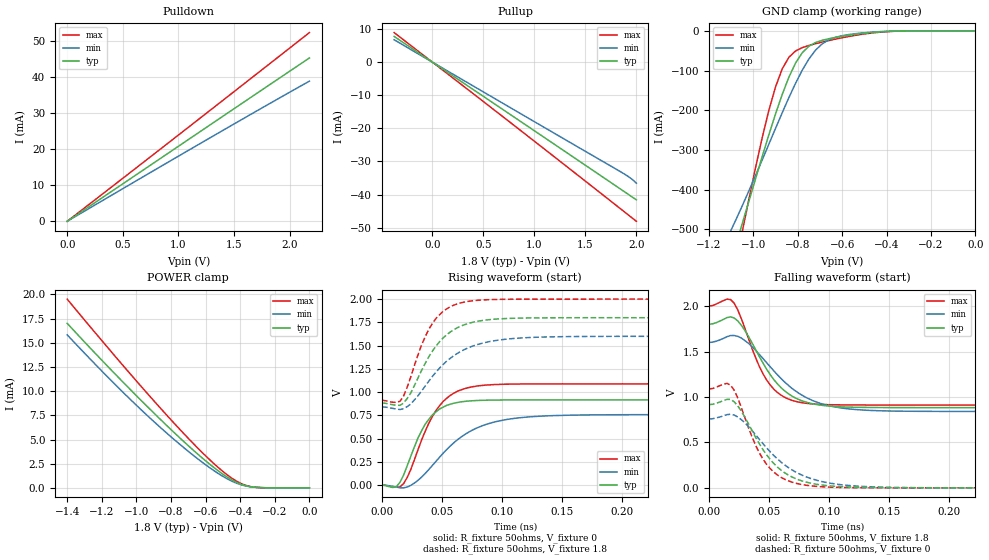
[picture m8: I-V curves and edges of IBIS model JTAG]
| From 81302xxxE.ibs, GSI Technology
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[Model]   JTAG
Model_type   Output
Polarity   Non-Inverting
Vmeas =   0.90v
Rref  =   50
|  variable   typ   min   max
C_comp   3.0pF   2.5pF   3.5pF
|  variable   typ   min   max
[Temperature Range]   50   100   0
|  variable   typ   min   max
[Voltage Range]   1.8   1.6   2.0
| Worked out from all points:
|   slope of the pulldown table from 0 to 0.27 V, typ, clamps not added: 48.2 ohm
|   slope of the pullup table from 0 to 0.27 V, typ, clamps not added: 48.4 ohm
|   GND clamp passes 1 mA (typ) near -0.37 V on its own axis
|   POWER clamp passes 1 mA (typ) near -0.46 V on its own axis
|   rising waveform, R_fixture 50ohms, V_fixture 0: 20-80 % time 20.3ps typ, 39.8ps min, 23.7ps max; typ from 0 V to 0.916 V
|   rising waveform, R_fixture 50ohms, V_fixture 1.8: 20-80 % time 27.1ps typ, 35.3ps min, 21.4ps max; typ from 0.883 V to 1.8 V
|   falling waveform, R_fixture 50ohms, V_fixture 1.8: 20-80 % time 28.2ps typ, 37.8ps min, 22ps max; typ from 1.8 V to 0.883 V
|   falling waveform, R_fixture 50ohms, V_fixture 0: 20-80 % time 29.5ps typ, 38.2ps min, 23.4ps max; typ from 0.916 V to 0 V
[Pullup]
| V(VDDQ-Vout)   typ   min   max
-376mV    7.795mA    6.799mA    8.961mA
1.856V    -38.6mA    -33.32mA   -44.6mA
1.952V    -40.61mA   -35.26mA   -46.93mA
2V        -41.61mA   -36.59mA   -48.1mA
[PullDown]
| voltage   typ   min   max
0V        -468.1pA   -1.371nA   -475.7pA
1.298V    26.99mA    23.38mA    31.07mA
1.782V    37.06mA    31.95mA    42.74mA
2.178V    45.27mA    38.85mA    52.3mA
[POWER Clamp]
|V(VDDQ-Vout)   typ   min   max
-1.4V     17.01mA    15.82mA    19.52mA
-1.12V    11.72mA    10.64mA    13.55mA
-868mV    7.194mA    6.351mA    8.377mA
-756mV    5.281mA    4.603mA    6.181mA
-644mV    3.468mA    2.981mA    4.09mA
-560mV    2.214mA    1.879mA    2.634mA
-476mV    1.125mA    943.2uA    1.354mA
-392mV    354.3uA    301.3uA    421.7uA
-336mV    105.8uA    97.24uA    116.6uA
-252mV    9.889uA    11.65uA    8.103uA
0V        25.53nA    51.16nA    8.026nA
[GND Clamp]
|(Vout)   typ   min   max
-1.5V     -1.208A    -946.4mA   -1.65A
-1.11V    -596.4mA   -513.8mA   -674.9mA
-1.08V    -541.5mA   -477.8mA   -590.3mA
-1.05V    -485.7mA   -440.9mA   -506.4mA
-930mV    -261.7mA   -285.3mA   -200mA
-900mV    -209.2mA   -245.6mA   -141mA
-870mV    -160.2mA   -206.3mA   -95.9mA
-810mV    -81.18mA   -132.2mA   -50.82mA
-720mV    -29.52mA   -48.7mA    -32.45mA
-630mV    -16.73mA   -16.29mA   -20.93mA
-390mV    -1.457mA   -1.082mA   -1.795mA
0V        -4.952nA   -11.78nA   -5.759nA
[Ramp]
| voltage   typ   min   max
dV/dt_r   0.54/186p   0.48/213p   0.60/209p
dV/dt_f   0.86/129p   0.66/166p   1.07/101p
R_load  =   50ohms
[Rising Waveform]
R_fixture =   50ohms
V_fixture =   0
| Time   V(typ)   V(min)   V(max)
0s        11.49nV    35.98nV    10.87nV
12ps      -17.48mV   -22.43mV   -22.97mV
18ps      107.4mV    -30.34mV   15.43mV
30ps      507.5mV    51.21mV    380.8mV
42ps      755.2mV    211.1mV    737.5mV
54ps      857.6mV    383.6mV    934.5mV
69ps      899.8mV    543.9mV    1.038V
93ps      914mV      675.8mV    1.08V
123ps     915.9mV    733.5mV    1.088V
297ps     916.1mV    757.6mV    1.089V
[Rising Waveform]
R_fixture =   50ohms
V_fixture =   1.8
V_fixture_min =  1.6
V_fixture_max =  2.0
| Time   V(typ)   V(min)   V(max)
0s        882.7mV    840.8mV    911.3mV
15ps      857.5mV    812.5mV    901.2mV
24ps      991.4mV    872.5mV    1.166V
33ps      1.234V     1.013V     1.508V
39ps      1.38V      1.118V     1.676V
51ps      1.584V     1.298V     1.87V
63ps      1.694V     1.418V     1.951V
84ps      1.771V     1.528V     1.991V
114ps     1.796V     1.581V     1.999V
297ps     1.8V       1.6V       2V
[Falling Waveform]
R_fixture =   50ohms
V_fixture =   1.8
V_fixture_min = 1.6
V_fixture_max = 2.0
| Time   V(typ)   V(min)   V(max)
0s        1.8V       1.6V       2V
15ps      1.873V     1.663V     2.077V
21ps      1.869V     1.676V     2.032V
30ps      1.731V     1.62V      1.753V
48ps      1.306V     1.378V     1.188V
60ps      1.103V     1.204V     1.02V
72ps      989.2mV    1.068V     952.1mV
93ps      910.1mV    928.7mV    918.5mV
123ps     886.4mV    860.9mV    912mV
297ps     882.7mV    840.8mV    911.3mV
[Falling Waveform]
R_fixture =   50ohms
V_fixture =   0
| Time   V(typ)   V(min)   V(max)
0s        916.1mV    757.7mV    1.089V
18ps      973.7mV    810mV      1.13V
27ps      844mV      750mV      880.7mV
36ps      628mV      628.9mV    557.2mV
45ps      420.6mV    486.5mV    316.6mV
57ps      229.1mV    319.1mV    142.3mV
72ps      102.9mV    176.1mV    52.11mV
96ps      28.13mV    63.88mV    10.78mV
126ps     5.678mV    17.47mV    1.591mV
297ps     25.21uV    38.27uV    23.83uV
